FUNCTION_BLOCK FB_AddProduct
VAR_IN_OUT
	fbClient:FB_IotHttpClient;
END_VAR
VAR_OUTPUT
	bBusy:BOOL;
	bError:BOOL;
	
END_VAR
VAR
	fbRequest			: FB_IotHttpRequest;
	fbJsonSend				: FB_JsonDomParser;
	jsonDoc				: SJsonValue;
	nState				: UDINT;
	AddRisingEdge			: R_TRIG;
	fbGetProductByBarCode:FB_GetProductByBarCode;
//	domParse:FB_JsonDomParser;
	
END_VAR
//HMI
VAR
	bSend:BOOL;
	nStatusCode:UINT;
	newProductBarCode:STRING[13];
	newProduct:ST_Product;
END_VAR

AddRisingEdge(CLK:=bSend , Q=> );
CASE nState OF
	0:
		IF AddRisingEdge.Q AND newProductBarCode<>'' THEN
			nStatusCode:=0;
			nState:=10;
			bBusy:=TRUE;
			bError:=FALSE;
		END_IF
	
	10:
		
		jsonDoc:=fbJsonSend.NewDocument();
		fbJsonSend.AddInt64Member(jsonDoc,'id',0);
		fbJsonSend.AddStringMember(jsonDoc,'barCode',newProductBarCode);
		fbJsonSend.AddDoubleMember(jsonDoc,'finalPressure',newProduct.FinalPressure);
		fbJsonSend.AddDoubleMember(jsonDoc,'finalDisplacement',newProduct.FinalDisplacement);
		fbJsonSend.AddBoolMember(jsonDoc,'isQualified',newProduct.IsQualified);
		IF fbRequest.SendJsonDomRequest(sUri:='/Product',fbClient:=fbClient,eRequestType:=ETcIotHttpRequestType.HTTP_POST,fbJson:=fbJsonSend,0) THEN
			nState:=20;
		END_IF
	20:
		IF NOT fbRequest.bBusy THEN
			nStatusCode:=fbRequest.nStatusCode;
			IF nStatusCode=200 THEN
				newProductBarCode:='';
			END_IF
			nState:=100;
		END_IF
			
	100:
		bBusy:=FALSE;
		nState:=0;
END_CASE

END_FUNCTION_BLOCK
